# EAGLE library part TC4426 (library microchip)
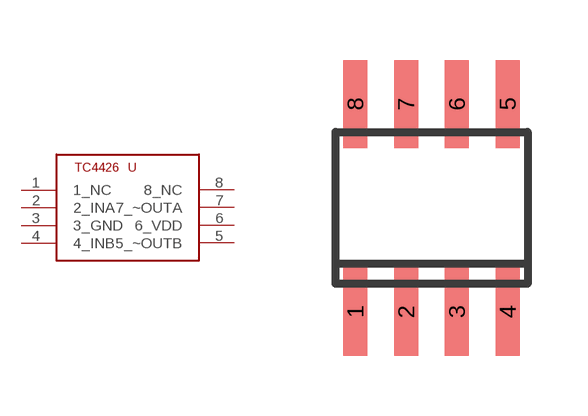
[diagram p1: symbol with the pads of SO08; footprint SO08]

Designator prefix -

## TC4426  [SO08]
1  1_NC
2  2_INA
3  3_GND
4  4_INB
5  5_~OUTB
6  6_VDD
7  7_~OUTA
8  8_NC

## Footprint SO08 (pad centres in mm)
Small Outline Package
smd 0.6 x 2.2: 1 -1.905,-2.6; 2 -0.635,-2.6; 3 0.635,-2.6; 4 1.905,-2.6; 5 1.905,2.6; 6 0.635,2.6; 7 -0.635,2.6; 8 -1.905,2.6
